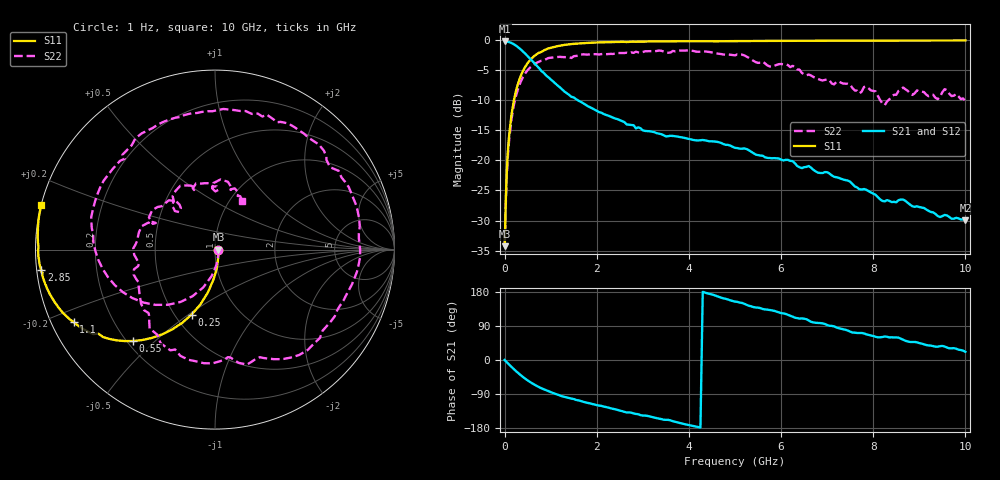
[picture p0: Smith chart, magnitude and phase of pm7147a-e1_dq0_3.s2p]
# GHz S DB R 50
! S-Parameters data
! Freq  dbS11  angS11  dbS21  angS21  dbS12  angS12  dbS22  angS22
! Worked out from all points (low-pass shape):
!   279 points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, 1 Hz to 10 GHz, reference 50 ohm
!   highest |S21| = -0.17 dB at 19.95 kHz (marker M1); lowest = -30.0 dB at 10 GHz (marker M2)
!   |S21| within 3 dB of the highest: start of sweep to 568.7 MHz
!   lowest |S11| = -34.3 dB at 19.95 kHz (marker M3), VSWR 1.04, Z = 52 - j0.00318 ohm
!   |S11| at or under -10 dB: start of sweep to 200.7 MHz
!   |S22| runs from -34.3 to -1.7 dB; largest |S21 - S12| = 0
!   S11 on the Smith chart (normalised r, x): 1 Hz: 1.04, -0.00; 250 MHz: 0.61, -0.51; 550 MHz: 0.22, -0.43; 1.1 GHz: 0.06, -0.24; 2.85 GHz: 0.01, -0.06; 10 GHz: 0.00, +0.12
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1e-09  -34.27 -0.0  -0.17 -0.0  -0.17 -0.0  -34.27 -0.0
1.99526e-05  -34.27 -0.1  -0.17 -0.0  -0.17 -0.0  -34.27 -0.1
0.03981072  -23.30 -77.0  -0.19 -4.9  -0.19 -4.9  -23.98 -77.8
0.07943282  -17.63 -89.0  -0.25 -9.8  -0.25 -9.8  -18.34 -92.8
0.25  -8.31 -109.7  -0.89 -29.7  -0.89 -29.7  -9.15 -123.3
0.55  -3.30 -131.8  -3.02 -57.9  -3.02 -57.9  -4.54 -160.5
1.1  -1.06 -152.9  -7.18 -89.3  -7.18 -89.3  -2.80 154.8
1.7  -0.47 -163.7  -10.44 -110.0  -10.44 -110.0  -2.32 122.2
2.85  -0.23 -173.3  -14.66 -142.3  -14.66 -142.3  -1.88 69.0
3.35  -0.16 -176.0  -15.54 -154.5  -15.54 -154.5  -1.69 45.3
4.3  -0.12 -179.9  -16.59 179.8  -16.59 179.8  -1.84 -0.2
5.05  -0.11 177.9  -17.93 153.5  -17.93 153.5  -2.33 -40.1
5.3  -0.11 177.2  -18.29 143.1  -18.29 143.1  -2.90 -58.5
6  -0.08 175.2  -19.85 123.8  -19.85 123.8  -3.93 -95.5
6.4  -0.06 174.2  -21.13 109.3  -21.13 109.3  -4.87 -129.7
6.7  -0.06 173.5  -21.56 99.2  -21.56 99.2  -6.08 -147.1
7.55  -0.03 171.3  -23.92 72.5  -23.92 72.5  -7.96 157.9
8.35  -0.02 169.4  -26.74 59.6  -26.74 59.6  -9.81 135.2
8.65  -0.02 168.7  -26.52 53.4  -26.52 53.4  -7.86 118.4
9.4  -0.01 167.1  -29.26 35.1  -29.26 35.1  -9.79 89.7
9.55  -0.01 166.7  -29.08 35.5  -29.08 35.5  -8.12 85.4
10  -0.01 165.8  -29.96 21.7  -29.96 21.7  -10.16 60.7
